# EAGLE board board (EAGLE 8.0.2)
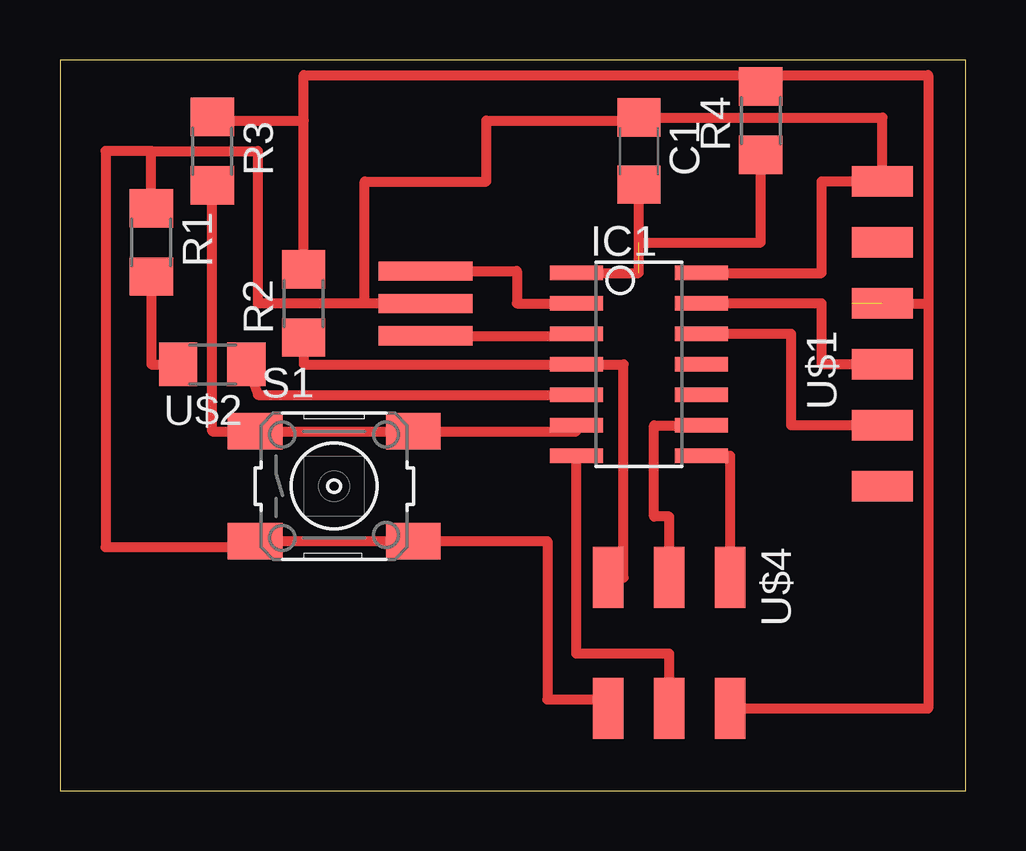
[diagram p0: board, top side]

Size 37.77 x 30.47 mm. Coordinates in mm from the lower left corner, seen from the top.
Outline: 0,0 37.77,0 37.77,30.47 0,30.47 0,0
Copper layers (1*16): Top 0.035mm / dielectric 1.5mm / Bottom 0.035mm
Design rules "default": minimum track width 10mil, minimum drill 24mil, track to track 8mil, track to pad 8mil, pad to pad 8mil, via to via 8mil, smd to smd 8mil, copper to edge 40mil, drill to drill 8mil, minimum pad ring 10mil, minimum via ring 8mil, stop-mask expansion 4mil, vias tented up to drill 0mil, thermal gap 10mil
Net classes: 0 default: width 0.35 mm, drill 0.4 mm, clearance 0.4 mm

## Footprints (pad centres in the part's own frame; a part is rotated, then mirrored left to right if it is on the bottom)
C1206 = smd 1.6 x 1.8: 1 -1.4,0; 2 1.4,0
SOIC14 = smd 0.61 x 2.21: 1 -3.81,-2.603; 2 -2.54,-2.603; 3 -1.27,-2.603; 4 0,-2.603; 5 1.27,-2.603; 6 2.54,-2.603; 7 3.81,-2.603; 8 3.81,2.603; 9 2.54,2.603; 10 1.27,2.603; 11 0,2.603; 12 -1.27,2.603; 13 -2.54,2.603; 14 -3.81,2.603
R1206 = smd 1.6 x 1.803: 1 -1.422,0; 2 1.422,0
6MM_SWITCH = smd 2.286 x 1.524: 1 -3.302,2.286; 2 3.302,2.286; 3 -3.302,-2.286; 4 3.302,-2.286
1X06SMD = smd 2.54 x 1.27: 1 0,6.35; 2 0,3.81; 3 0,1.27; 4 0,-1.27; 5 0,-3.81; 6 0,-6.35
LED1206 = smd 1.6 x 1.803: 1 -1.422,0; 2 1.422,0
EFOBM = smd 0.8 x 3.9: 1 -1.35,0; 2 0,0; 3 1.35,0
2X03SMD = smd 2.54 x 1.27: 1 -2.54,2.54; 2 2.92,2.54; 3 -2.54,0; 4 2.92,0; 5 -2.54,-2.54; 6 2.92,-2.54

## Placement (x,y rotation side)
C1  [C1206]  24.13,26.67 270 top
IC1  ATTINY44-SSU  [SOIC14]  24.13,17.78 270 top
R1  [R1206]  3.81,22.86 270 top
R2  [R1206]  10.16,20.32 90 top
R3  [R1206]  6.35,26.67 270 top
R4  [R1206]  29.21,27.94 90 top
S1  [6MM_SWITCH]  11.43,12.7 0 top
U$1  FTDI-SMD-HEADER  [1X06SMD]  34.29,19.05 0 top
U$2  LED  [LED1206]  6.35,17.78 180 top
U$3  RESONATOR  [EFOBM]  15.24,20.32 270 top
U$4  AVRISPSMD  [2X03SMD]  25.4,6.35 270 top

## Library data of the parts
C1 IC1 R1-R4 S1 U$1-U$4 = fab

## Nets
GND: C1.1 IC1.14 R1.1 S1.3 S1.4 U$1.1 U$3.2 U$4.6
MOSI: IC1.7 U$4.4
N$1: IC1.8 U$4.1
N$3: IC1.13 U$1.4
N$4: IC1.12 U$1.5
N$5: IC1.9 U$4.3
N$6: IC1.2 U$3.1
N$7: IC1.3 U$3.3
N$8: IC1.5 U$2.1
N$9: R1.2 U$2.2
N$10: IC1.6 R3.2 S1.1 S1.2
N$11: IC1.4 R2.1 U$4.5
VCC: C1.2 IC1.1 R2.2 R3.1 U$1.3 U$4.2

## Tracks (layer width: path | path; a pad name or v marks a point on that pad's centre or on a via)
GND
  Top 0.406: U$3.2 12.7,20.32 | 12.7,20.32 8.26,20.32 8.26,26.67 3.81,26.67 | 3.81,26.67 1.91,26.67 1.91,10.16 8.13,10.16 S1.3 S1.4 20.32,10.41 20.32,3.81 22.86,3.81 U$4.6 | R1.1 3.81,26.67 | 12.7,20.32 12.7,25.4 17.78,25.4 17.78,27.94 24.13,27.94 C1.1 34.29,28.07 U$1.1 31.75,25.4 31.75,21.59 IC1.14
MOSI
  Top 0.406: U$4.4 25.4,5.71 21.53,5.71 IC1.7
N$1
  Top 0.406: U$4.1 27.94,13.97 IC1.8
N$3
  Top 0.406: U$1.4 31.75,17.78 31.75,20.32 IC1.13
N$4
  Top 0.406: U$1.5 30.48,15.24 30.48,19.05 IC1.12
N$5
  Top 0.406: U$4.3 25.4,11.43 24.77,11.43 24.77,15.24 IC1.9
N$6
  Top 0.406: U$3.1 19.05,21.67 19.05,20.32 IC1.2
N$7
  Top 0.406: U$3.3 21.53,18.97 IC1.3
N$8
  Top 0.406: U$2.1 8.26,16.51 IC1.5
N$9
  Top 0.406: R1.2 3.81,17.78 U$2.2
N$10
  Top 0.406: IC1.6 21.53,14.99 S1.2 S1.1 6.35,14.99 R3.2
N$11
  Top 0.406: U$4.5 23.49,8.89 23.49,17.78 IC1.4 10.16,17.78 R2.1
VCC  (2 unrouted)
  Top 0.406: U$4.2 36.2,3.43 36.2,20.32 | U$1.3 36.2,20.32 | R3.1 6.35,27.94 10.16,27.94 | R2.2 10.16,27.94 | IC1.1 24.13,21.59 C1.2 | 10.16,27.94 10.16,29.84 36.2,29.84 36.2,20.32 | 24.13,22.86 29.21,22.86 29.21,26.67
